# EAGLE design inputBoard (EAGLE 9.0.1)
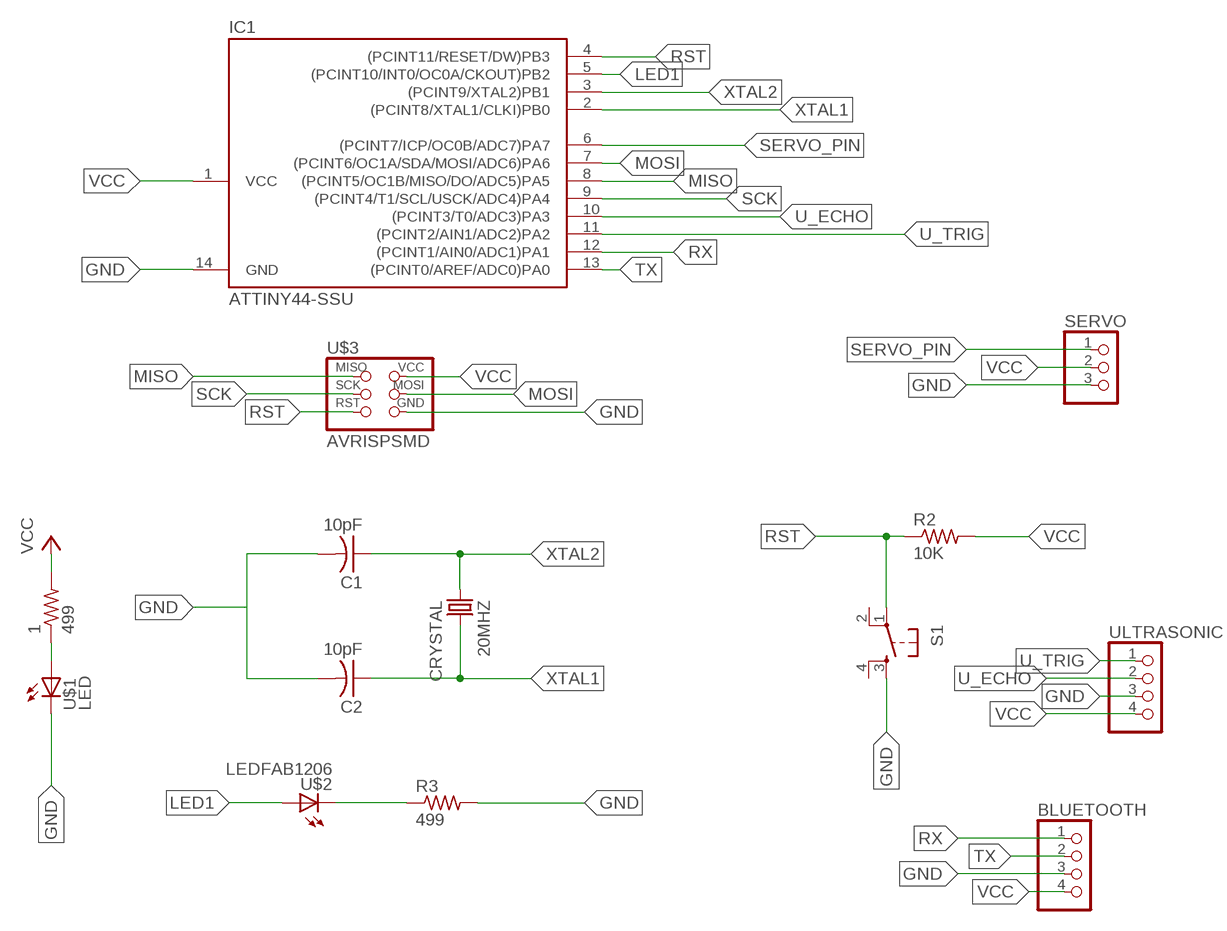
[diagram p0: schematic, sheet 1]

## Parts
1  499  RES-US1206FAB  [R1206FAB]
20MHZ  CRYSTAL  [2-SMD-5X3MM]
BLUETOOTH  PINHD-1X4  [1X04]
C1  10pF  CAP-US1206FAB  [C1206FAB]
C2  10pF  CAP-US1206FAB  [C1206FAB]
IC1  ATTINY44-SSU  [SOIC14]
R2  10K  RES-US1206FAB  [R1206FAB]
R3  499  RES-US1206FAB  [R1206FAB]
S1  6MM_SWITCH6MM_SWITCH  [6MM_SWITCH]
SERVO  PINHD-1X3  [1X03]
U$1  LED  [LED1206]
U$2  LEDFAB1206  [LED1206FAB]
U$3  AVRISPSMD  [2X03SMD]
ULTRASONIC  PINHD-1X4  [1X04]

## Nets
GND: BLUETOOTH.3 C1.2 C2.2 IC1.14(GND) R3.2 S1.3(S) SERVO.3 U$1.2(C) U$3.6(GND) ULTRASONIC.3
LED1: IC1.5((PCINT10/INT0/OC0A/CKOUT)PB2) U$2.1(A)
MISO: IC1.8((PCINT5/OC1B/MISO/DO/ADC5)PA5) U$3.1(MISO)
MOSI: IC1.7((PCINT6/OC1A/SDA/MOSI/ADC6)PA6) U$3.4(MOSI)
N$1: R3.1 U$2.2(C)
N$2: 1.1 U$1.1(A)
RST: IC1.4((PCINT11/RESET/DW)PB3) R2.1 S1.1(P) U$3.5(RST)
RX: BLUETOOTH.1 IC1.12((PCINT1/AIN0/ADC1)PA1)
SCK: IC1.9((PCINT4/T1/SCL/USCK/ADC4)PA4) U$3.3(SCK)
SERVO_PIN: IC1.6((PCINT7/ICP/OC0B/ADC7)PA7) SERVO.1
TX: BLUETOOTH.2 IC1.13((PCINT0/AREF/ADC0)PA0)
U_ECHO: IC1.10((PCINT3/T0/ADC3)PA3) ULTRASONIC.2
U_TRIG: IC1.11((PCINT2/AIN1/ADC2)PA2) ULTRASONIC.1
VCC: 1.2 BLUETOOTH.4 IC1.1(VCC) R2.2 SERVO.2 U$3.2(VCC) ULTRASONIC.4
XTAL1: 20MHZ.P$2 C2.1 IC1.2((PCINT8/XTAL1/CLKI)PB0)
XTAL2: 20MHZ.P$1 C1.1 IC1.3((PCINT9/XTAL2)PB1)
Unconnected: S1.2(P1) S1.4(S1)

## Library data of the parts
1 R2 R3 = fab:RES-US: Resistor (US Symbol)
20MHZ = fab:CRYSTAL
BLUETOOTH ULTRASONIC = pinhead:PINHD-1X4: PIN HEADER
C1 C2 = fab:CAP-US
IC1 = fab:ATTINY44
S1 = fab:6MM_SWITCH: OMRON SWITCH
SERVO = pinhead:PINHD-1X3: PIN HEADER
U$1 U$2 = fab:LED: LED
U$3 = fab:AVRISP

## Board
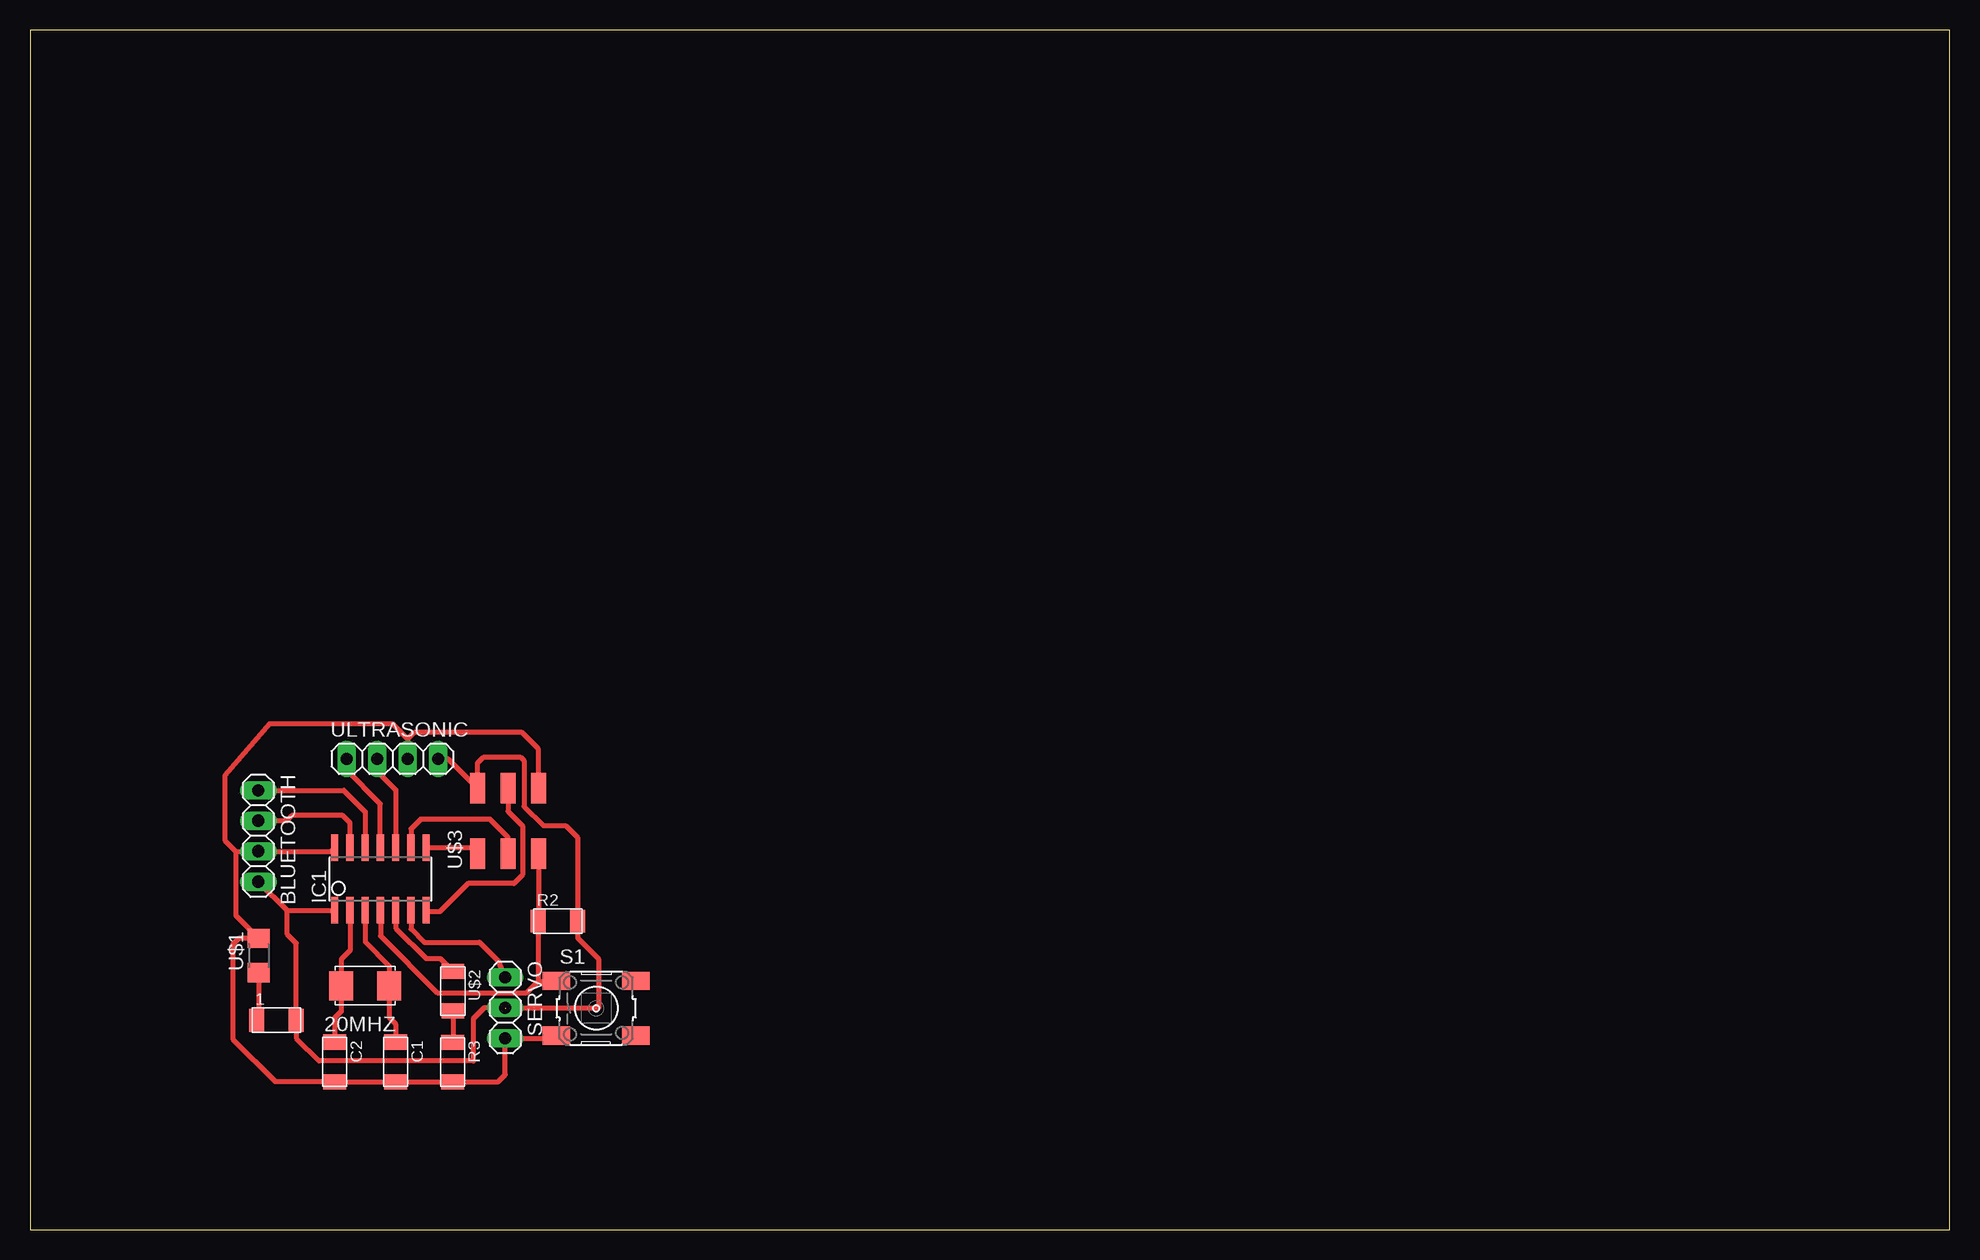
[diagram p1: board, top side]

Size 160 x 100 mm. Coordinates in mm from the lower left corner, seen from the top.
Outline: 0,0 160,0 160,100 0,100 0,0
Copper layers (1*16): Top 0.035mm / dielectric 1.5mm / Bottom 0.035mm
Design rules "default": minimum track width 6mil, minimum drill 0.35mm, track to track 6mil, track to pad 6mil, pad to pad 6mil, via to via 6mil, smd to smd 6mil, copper to edge 40mil, drill to drill 6mil, minimum pad ring 10mil, minimum via ring 8mil, stop-mask expansion 4mil, vias tented up to drill 0mil, thermal gap 10mil

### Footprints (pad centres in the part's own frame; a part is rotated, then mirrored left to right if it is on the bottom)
R1206FAB = smd 1.27 x 1.905: 1 -1.651,0; 2 1.651,0
2-SMD-5X3MM = smd 2 x 2.4: P$1 -2,0; P$2 2,0
1X04 = drill 1.016 long: 1 -3.81,0; 2 -1.27,0; 3 1.27,0; 4 3.81,0
C1206FAB = smd 1.27 x 1.905: 1 -1.651,0; 2 1.651,0
SOIC14 = smd 0.61 x 2.21: 1 -3.81,-2.603; 2 -2.54,-2.603; 3 -1.27,-2.603; 4 0,-2.603; 5 1.27,-2.603; 6 2.54,-2.603; 7 3.81,-2.603; 8 3.81,2.603; 9 2.54,2.603; 10 1.27,2.603; 11 0,2.603; 12 -1.27,2.603; 13 -2.54,2.603; 14 -3.81,2.603
6MM_SWITCH = smd 2.286 x 1.524: 1 -3.302,2.286; 2 3.302,2.286; 3 -3.302,-2.286; 4 3.302,-2.286
1X03 = drill 1.016 long: 1 -2.54,0; 2 0,0; 3 2.54,0
LED1206 = smd 1.6 x 1.803: 1 -1.422,0; 2 1.422,0
LED1206FAB = smd 1.27 x 1.905: 1 -1.651,0; 2 1.651,0
2X03SMD = smd 2.54 x 1.27: 1 -2.54,2.54; 2 2.92,2.54; 3 -2.54,0; 4 2.92,0; 5 -2.54,-2.54; 6 2.92,-2.54

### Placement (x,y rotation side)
1  20.54,17.45 0 top
20MHZ  27.94,20.32 180 top
BLUETOOTH  19.03,32.81 270 top
C1  30.48,13.97 270 top
C2  25.4,13.97 270 top
IC1  29.21,29.21 0 top
R2  44.01,25.71 0 top
R3  35.23,13.95 270 top
S1  47.19,18.45 0 top
SERVO  39.61,18.49 270 top
U$1  19.07,22.84 90 top
U$2  35.26,19.88 270 top
U$3  39.85,33.85 90 top
ULTRASONIC  30.21,39.23 0 top

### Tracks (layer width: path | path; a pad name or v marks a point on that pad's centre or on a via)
GND
  Top 0.406: IC1.14 25.12,31.54 BLUETOOTH.3 17.16,31.54 | 17.16,31.54 16.24,32.46 16.24,37.84 19.96,42.18 30.2,42.18 31.48,40.9 | 31.48,40.9 ULTRASONIC.3 | U$3.6 42.39,40.05 41.03,41.42 32.01,41.42 31.48,40.9 | 17.16,31.54 17.16,29.47 17.15,29.46 17.15,26.18 U$1.2 17.39,24.26 16.91,23.77 16.91,15.86 20.42,12.35 25.37,12.35 C2.2 C1.2 35.21,12.32 R3.2 39.01,12.3 39.61,12.9 SERVO.3 43.68,15.95 S1.3
LED1
  Top 0.406: IC1.5 30.48,25.12 33.01,22.59 34.19,22.59 U$2.1
MISO
  Top 0.406: U$3.1 36.81,31.81 IC1.8
MOSI
  Top 0.406: IC1.7 33.13,26.49 34.15,26.49 36.51,28.85 40.34,28.85 41.05,29.56 41.05,33.67 39.85,34.86 U$3.4
N$1
  Top 0.406: U$2.2 35.26,15.63 R3.1
N$2
  Top 0.406: U$1.1 19.07,17.62 1.1
RST
  Top 0.406: IC1.4 29.21,24.47 33.94,19.74 41.4,19.74 42.35,20.7 | U$3.5 42.39,25.75 R2.1 42.35,20.7 | 42.35,20.7 S1.1
RX
  Top 0.406: BLUETOOTH.1 26.15,36.62 27.94,34.82 IC1.12
SCK
  Top 0.406: U$3.3 39.85,32.71 38.36,34.2 32.54,34.2 31.75,33.41 IC1.9
SERVO_PIN
  Top 0.406: IC1.6 31.75,25.04 32.85,23.95 37.48,23.95 38.91,22.51 38.96,22.43 SERVO.1
TX
  Top 0.406: IC1.13 26.67,33.91 26.08,34.5 21.83,34.5 21.4,34.08 BLUETOOTH.2
U_ECHO
  Top 0.406: IC1.10 30.48,36.66 28.94,38.2 ULTRASONIC.2
U_TRIG
  Top 0.406: IC1.11 29.19,31.83 29.19,35.5 26.4,38.29 ULTRASONIC.1
VCC  (1 unrouted)
  Top 0.406: BLUETOOTH.4 21.42,26.61 21.44,26.61 | 21.44,26.61 IC1.1 | 21.44,26.61 21.44,24.62 22.19,23.87 1.2 22.19,15.95 24.09,14.05 36.95,14.05 36.95,17.56 37.87,18.49 SERVO.2 | 39.65,18.45 47.38,18.45 47.38,22.58 45.66,24.3 R2.2 45.64,25.73 45.64,32.67 44.64,33.67 42.8,33.67 41.19,35.28 41.19,39.09 40.89,39.38 37.82,39.38 37.31,38.88 U$3.2 34.85,39.23 ULTRASONIC.4
XTAL1
  Top 0.406: IC1.2 26.67,23.27 25.94,22.54 20MHZ.P$2 25.94,18.18 25.41,17.66 25.41,15.63 C2.1
XTAL2
  Top 0.406: IC1.3 27.95,23.96 29.95,21.95 20MHZ.P$1 29.94,17.69 30.46,17.17 30.46,15.64 C1.1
